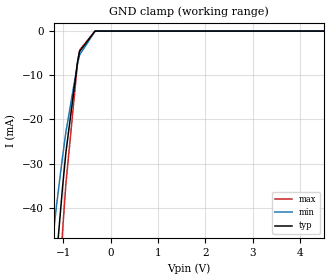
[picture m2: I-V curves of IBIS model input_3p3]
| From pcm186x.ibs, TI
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|   input_3p3 Model
[Model]   input_3p3
Model_type   Input
Vinl = 0.99
Vinh = 2.31
|   typ   min   max
|   (nom PVT)   (fast PVT)   (slow PVT)
C_comp   5.099e-12   5.099e-12   5.099e-12
[Model spec]
|subparameter
Vinl   0.99   0.9   1.08
Vinh   2.31   2.1   2.52
| Where nom  PVT is Nominal Process, 3.3V, 27C
|   Fast PVT is Strong Process,  3.6V, -40C
|   Slow PVT is Weak Process,   3V, 125C
[Voltage Range]   3.3   3   3.6
|Junction Temperature
[Temperature Range]   27   125   -40
[Power Clamp Reference]   3.3   3   3.6
[GND Clamp Reference]   0   0   0
[GND Clamp]
|   Voltage   I(typ)   I(min)   I(max)
-3.3V     -1.65A     -1.372A    -1.926A
-1.406V   -90.83mA   -66.27mA   -122.9mA
-1.169V   -54.85mA   -41.94mA   -72.53mA
-1.136V   -50.46mA   -38.92mA   -66.4mA
-1.013V   -35.05mA   -28.22mA   -44.97mA
-945mV    -27.5mA    -22.86mA   -34.55mA
-699mV    -6.951mA   -7.399mA   -7.185mA
-669.9mV  -5.349mA   -6.051mA   -5.221mA
-654mV    -4.563mA   -5.366mA   -4.284mA
-330mV    -3.565uA   -33.04uA   -355.6nA
6.6V      0A         0A         0A
[POWER Clamp]
|   Voltage   I(typ)   I(min)   I(max)
-3.3V     0A         0A         0A
0V        0A         0A         0A
6.6V      0A         0A         0A
